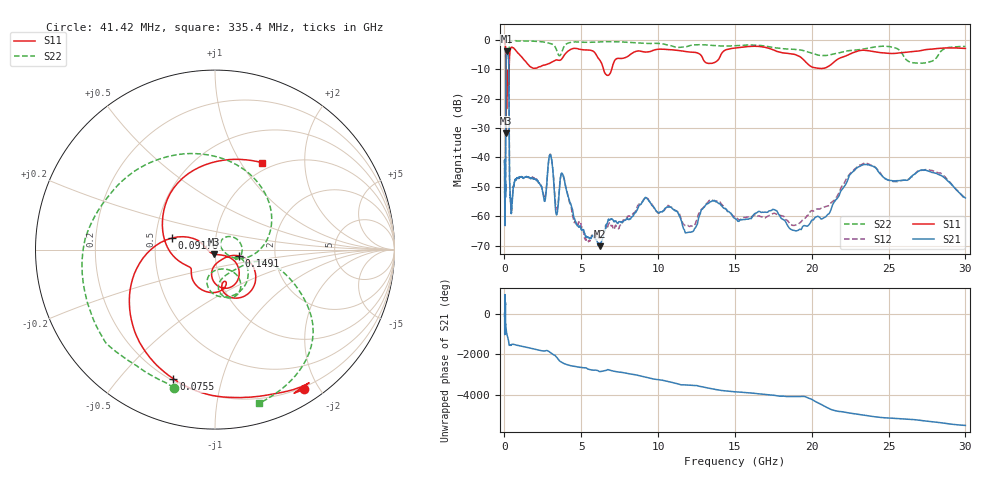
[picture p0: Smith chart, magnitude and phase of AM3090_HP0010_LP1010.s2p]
! Date/Time: Thu, Feb 28, 2019 1:55 PM
! Network Analyzer: Agilent Technologies E8364B Rev: A.07.50.67
! Sweep from 0.010 to 30.000 GHz, 1601 Points, Sweep Type: LOG
! Power Supply: 5.022 V, 0.002 A
# Hz S DB R 50
!freq MagS11 AngS11 MagS21 AngS21 MagS12 AngS12 MagS22 AngS22
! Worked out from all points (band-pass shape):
!   1601 points, 10 MHz to 30 GHz, reference 50 ohm
!   highest |S21| = -3.78 dB at 149.9 MHz (marker M1); lowest = -70.2 dB at 6.202 GHz (marker M2)
!   |S21| within 3 dB of the highest: 101.8 MHz to 270.5 MHz (168.7 MHz wide, 90.6 % of centre)
!   lowest |S11| = -31.8 dB at 99.92 MHz (marker M3), VSWR 1.05, Z = 49.2 - j2.41 ohm
!   |S11| at or under -10 dB: 90.66 MHz to 298.3 MHz (207.6 MHz wide, 107 % of centre); 6.452 GHz to 6.979 GHz (527.8 MHz wide, 7.86 % of centre)
!   |S22| runs from -29.0 to -0.2 dB; largest |S21 - S12| = 0.017
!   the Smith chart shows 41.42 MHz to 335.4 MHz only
!   S11 on the Smith chart (normalised r, x): 41.42 MHz: 0.17, -1.81; 75.5 MHz: 0.21, -0.71; 91.78 MHz: 0.61, +0.08; 149.1 MHz: 1.31, -0.09; 335.4 MHz: 0.90, +1.25
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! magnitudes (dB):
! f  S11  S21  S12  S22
! 10 MHz  -0.2  -41.7  -40.9  -0.6
! 38.04 MHz  -0.5  -61.4  -61.2  -1.6
! 41.42 MHz  -0.7  -60.3  -60.1  -1.9
! 75.5 MHz  -2.4  -48.2  -46.3  -4.5
! 91.78 MHz  -12.1  -14.7  -14.7  -11.9
! 99.92 MHz  -31.8  -7.4  -7.4  -28.1
! 115.5 MHz  -13.1  -4.9  -4.9  -18.1
! 144.7 MHz  -21.1  -3.8  -3.8  -18.4
! 149.1 MHz  -17.1  -3.8  -3.8  -17.3
! 149.9 MHz  -16.6  -3.8  -3.8  -17.1
! 274.6 MHz  -15.0  -7.4  -7.4  -16.2
! 335.4 MHz  -5.2  -47.9  -47.8  -1.0
! 550.5 MHz  -2.6  -51.3  -51.7  -0.3
! 2.084 GHz  -9.6  -47.8  -47.3  -0.5
! 2.987 GHz  -7.8  -39.1  -38.9  -1.2
! 3.385 GHz  -6.7  -59.6  -57.5  -3.3
! 3.779 GHz  -6.1  -45.6  -45.7  -3.4
! 6.202 GHz  -6.8  -70.2  -67.6  -0.6
! 7.926 GHz  -5.9  -61.0  -60.8  -0.8
! 19.22 GHz  -5.6  -64.4  -62.3  -3.4
! 23.48 GHz  -3.5  -42.4  -41.8  -3.0
! 30 GHz  -2.9  -53.8  -54.2  -2.2
